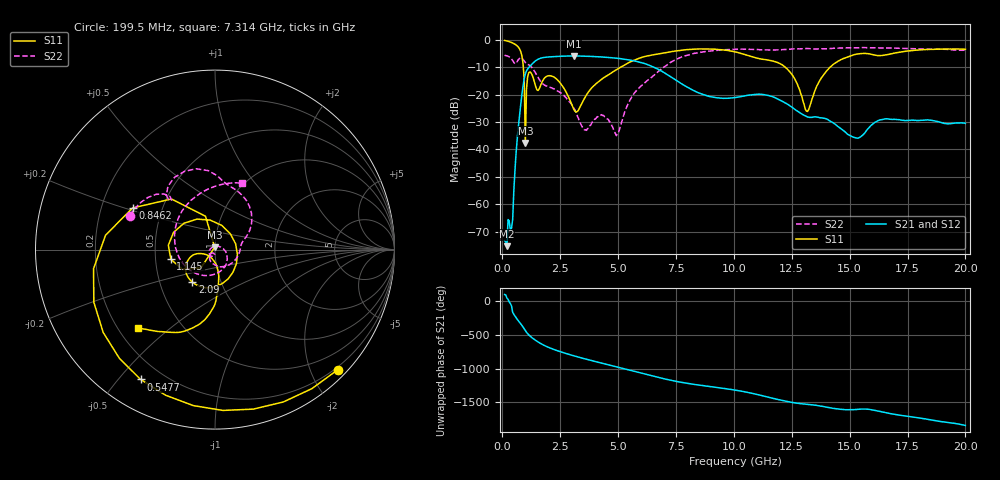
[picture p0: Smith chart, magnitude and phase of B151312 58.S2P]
!  2-Port S-parameters saved by WinCal
! VAR MeasName=S-Parameters (CALIBRATED_DATA) read from VNA (N5244A)
! VAR MeasDate=12/8/2015 5:48:19 PM
! VAR NAME=B151312 58
! VAR FILENAME=B151312 58.S2P
! VAR DATE=12/8/2015 5:48:20 PM
! VAR PHYS_PORTS=1,2
# Hz S DB R 50
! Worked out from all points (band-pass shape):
!   401 points, 100 MHz to 20 GHz, reference 50 ohm
!   highest |S21| = -5.84 dB at 3.085 GHz (marker M1); lowest = -75.3 dB at 199.5 MHz (marker M2)
!   |S21| within 3 dB of the highest: 1.281 GHz to 6.218 GHz (4.937 GHz wide, 132 % of centre)
!   lowest |S11| = -37.6 dB at 995.5 MHz (marker M3), VSWR 1.03, Z = 49.8 + j1.3 ohm
!   |S11| at or under -10 dB: 908.3 MHz to 5.105 GHz (4.196 GHz wide, 140 % of centre); 12.22 GHz to 14.15 GHz (1.928 GHz wide, 14.6 % of centre)
!   |S22| runs from -34.9 to -2.8 dB; largest |S21 - S12| = 0.0017
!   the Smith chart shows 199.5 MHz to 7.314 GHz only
!   S11 on the Smith chart (normalised r, x): 199.5 MHz: 0.15, -2.44; 547.8 MHz: 0.12, -0.57; 846.2 MHz: 0.34, +0.21; 1.145 GHz: 0.60, -0.07; 2.09 GHz: 0.73, -0.28; 7.314 GHz: 0.28, -0.39
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1e8  -0.20 -22.6  -73.28 99.8  -72.88 117.3  -5.63 169.3
1.995e8  -0.38 -44.4  -75.33 46.8  -71.68 39.0  -5.82 158.4
3.985e8  -0.94 -87.2  -68.79 -68.1  -67.98 -55.2  -6.94 136.8
5.4775e8  -1.58 -119.8  -47.58 140.5  -47.57 140.3  -8.71 131.1
8.4625e8  -5.77 153.2  -20.02 3.4  -20.01 3.4  -6.70 103.0
9.955e8  -37.63 97.6  -12.39 -74.5  -12.39 -74.5  -8.27 83.8
1.14475e9  -11.97 -167.5  -10.09 -138.2  -10.09 -138.2  -9.09 69.9
1.64225e9  -16.88 -33.9  -6.71 96.8  -6.71 96.8  -15.01 20.3
2.09e9  -13.12 -124.7  -6.17 23.9  -6.17 23.8  -17.41 -9.9
3.085e9  -25.33 -147.8  -5.84 -87.9  -5.85 -87.9  -24.77 -120.6
3.43325e9  -23.21 -91.6  -5.90 -121.0  -5.89 -121.0  -31.44 -134.3
4.1795e9  -15.07 -83.7  -6.18 172.9  -6.17 172.9  -27.59 -114.8
5.02525e9  -10.38 -90.0  -6.75 100.7  -6.75 100.7  -33.72 70.0
5.92075e9  -6.67 -107.4  -8.11 23.2  -8.08 23.1  -17.41 -88.2
6.7665e9  -5.08 -125.1  -10.88 -50.6  -10.87 -50.7  -11.32 137.8
7.31375e9  -4.26 -134.7  -13.67 -93.3  -13.64 -93.6  -7.97 68.2
8.3585e9  -3.34 -155.9  -18.90 -155.5  -18.87 -156.0  -4.80 -8.7
1.005e10  -4.36 168.4  -21.05 123.7  -21.06 123.2  -3.40 -69.8
1.338325e10  -21.42 -57.1  -28.28 -93.2  -28.30 -93.1  -3.27 -120.9
1.45275e10  -7.63 -115.2  -31.84 -158.1  -31.81 -158.6  -3.01 -131.1
1.67165e10  -5.24 -156.0  -28.95 137.8  -28.86 137.5  -2.93 -153.0
2e10  -3.41 163.1  -30.48 -40.6  -30.62 -41.2  -3.77 -176.7
